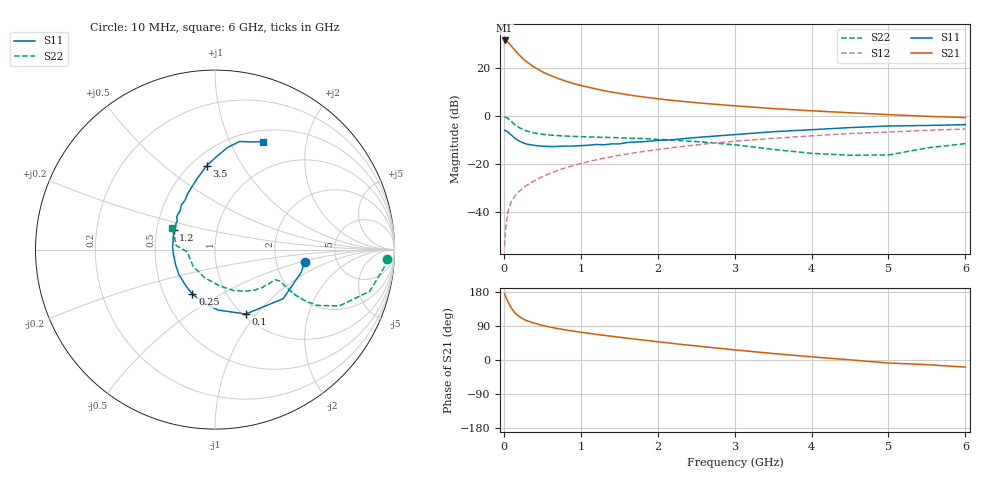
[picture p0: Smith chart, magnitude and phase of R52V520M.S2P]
! SIEMENS Small Signal Semiconductors
! BFR183
! Si NPN RF Bipolar Junction Transistor in SOT23
! VCE = 2.5 V  IC = 20 mA
! Common Emitter S-Parameters:  May  1996
# GHz  S  MA  R  50
!  f  S11  S21  S12  S22
! GHz  MAG  ANG  MAG  ANG  MAG  ANG  MAG  ANG
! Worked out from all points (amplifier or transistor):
!   36 points, 10 MHz to 6 GHz, reference 50 ohm
!   highest |S21| = 31.3 dB at 10 MHz (marker M1)
!   |S21| within 3 dB of that: start of sweep to 116 MHz
!   unconditionally stable (mu >= 1): 520.8 MHz to 2.383 GHz
!   at 250 MHz: K = 0.82, MSG = 26.8 dB, |S12| = -29.9 dB
!   at 1.4 GHz: K = 1.05, MAG = 12.0 dB, |S12| = -16.9 dB
!   at 6 GHz: K = 0.90, MSG = 2.4 dB, |S12| = -5.4 dB
!   S11 on the Smith chart (normalised r, x): 10 MHz: 2.93, -0.53; 100 MHz: 1.03, -0.88; 250 MHz: 0.69, -0.37; 1.2 GHz: 0.61, +0.14; 3.5 GHz: 0.59, +0.71; 6 GHz: 0.63, +1.34
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0.01  0.5042 -7.7  36.57 174.6  0.002 87.8  0.9597 -3.0
0.02  0.4972 -14.6  36.37 169.1  0.004 87.8  0.9459 -6.3
0.05  0.4679 -35.8  34 154.8  0.0099 75.5  0.8924 -15.1
0.1  0.3977 -64.5  27.77 136.2  0.0172 70.7  0.7601 -24.4
0.15  0.337 -87.2  22.31 123.0  0.0225 67.9  0.6492 -28.6
0.2  0.3009 -103.5  18.3 114.6  0.0274 68.4  0.5726 -29.6
0.25  0.2773 -117.0  15.27 108.3  0.0319 68.4  0.52 -29.5
0.3  0.26 -128.2  13.09 103.6  0.0367 68.8  0.4858 -29.0
0.4  0.2445 -145.3  10.15 96.9  0.0459 70.3  0.4412 -27.5
0.5  0.2357 -158.0  8.222 91.4  0.055 71.3  0.4154 -26.5
0.6  0.2319 -167.3  6.937 87.0  0.0644 71.3  0.4012 -26.0
0.7  0.2333 -175.3  6.003 83.1  0.0743 71.3  0.3911 -26.1
0.8  0.2368 177.0  5.27 79.5  0.0837 70.8  0.3828 -26.3
0.9  0.2372 171.0  4.711 76.3  0.0936 70.5  0.3763 -26.6
1.1  0.2467 159.4  3.92 70.6  0.1134 69.4  0.3674 -28.7
1.2  0.2561 154.5  3.614 67.8  0.123 68.8  0.3626 -29.6
1.6  0.2805 139.5  2.753 57.5  0.1617 64.8  0.3457 -35.1
2.2  0.3213 121.4  2.083 43.7  0.2212 58.6  0.3162 -45.6
3.5  0.4705 95.6  1.418 17.1  0.3429 42.0  0.2025 -83.2
4.5  0.5723 83.1  1.162 0.4  0.4309 29.2  0.1534 -142.6
5.5  0.6338 71.1  0.981 -12.2  0.5025 17.4  0.2168 174.1
6  0.6593 65.9  0.925 -18.8  0.5355 9.7  0.267 152.8
